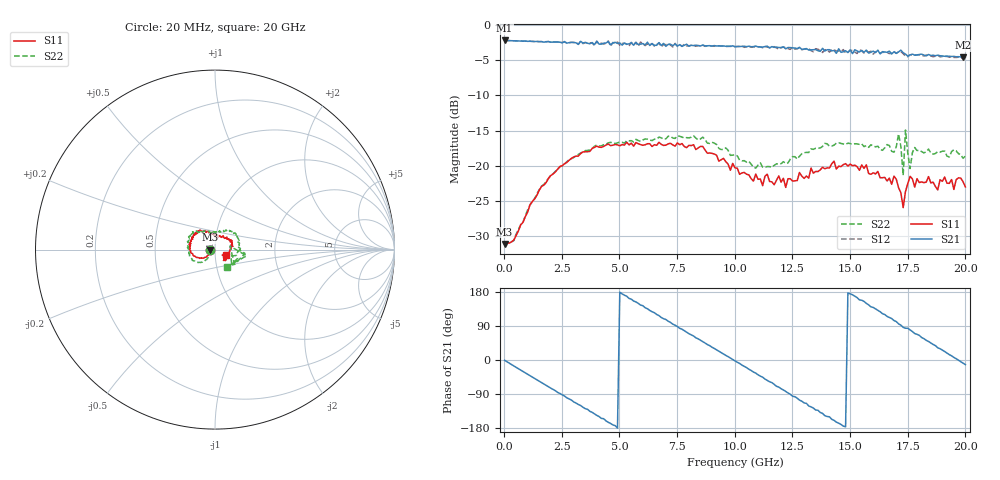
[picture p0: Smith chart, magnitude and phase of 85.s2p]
!Agilent Technologies,N5230A,US43500223,A.07.50.48
!Agilent N5230A: A.07.50.48
!Date: Saturday, September 19, 2015 17:07:46
!Correction: S11(Full 2 Port(1,2))
!S21(Full 2 Port(1,2))
!S12(Full 2 Port(1,2))
!S22(Full 2 Port(1,2))
!S2P File: Measurements: S11, S21, S12, S22:
# Hz S  RI  R 50
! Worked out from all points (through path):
!   201 points, 20 MHz to 20 GHz, reference 50 ohm
!   highest |S21| = -2.19 dB at 20 MHz (marker M1); lowest = -4.6 dB at 19.9 GHz (marker M2)
!   group delay of S21, straight-line fit = 101 ps
!   lowest |S11| = -31.1 dB at 20 MHz (marker M3), VSWR 1.06, Z = 47.3 - j0.034 ohm
!   |S11| at or under -10 dB: start of sweep to end of sweep
!   |S22| runs from -31.4 to -14.9 dB; largest |S21 - S12| = 0.057
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2e7  -0.0278 -0.000359  0.7774 -0.0112  0.7769 -0.0113  -0.0268 0.000192
1.8182e9  -0.0606 -0.0458  0.3007 -0.6992  0.2995 -0.7008  -0.0522 -0.0568
3.4166e9  -0.121 -0.0338  -0.4231 -0.6138  -0.4281 -0.6017  -0.1048 -0.0687
4.9151e9  -0.1398 0.0171  -0.7403 -0.0037  -0.7584 0.00662  -0.1438 -0.022
5.7143e9  -0.141 0.0386  -0.6715 0.3382  -0.6748 0.3387  -0.1536 0.012
6.7133e9  -0.129 0.0702  -0.342 0.6677  -0.346 0.662  -0.1535 0.0451
8.1119e9  -0.0984 0.0984  0.2876 0.6581  0.2739 0.6653  -0.1364 0.0826
9.1109e9  -0.0618 0.1044  0.6162 0.3624  0.6031 0.3704  -0.1016 0.1034
1.001e10  -0.0247 0.0933  0.7017 -0.0291  0.7021 -0.0167  -0.0611 0.1029
1.09091e10  -0.00581 0.0871  0.584 -0.4022  0.5836 -0.3874  -0.0137 0.0954
1.18082e10  0.0127 0.0779  0.2459 -0.6525  0.2617 -0.637  0.0158 0.102
1.34066e10  0.0627 0.0626  -0.3987 -0.5359  -0.3683 -0.5312  0.0828 0.1014
1.5005e10  0.0957 0.0374  -0.6622 0.0645  -0.6635 0.0286  0.1235 0.0735
1.67033e10  0.0791 -0.0205  -0.247 0.6043  -0.2574 0.5722  0.1392 -0.00276
1.71029e10  0.0605 -0.0348  -0.0608 0.642  -0.1018 0.6376  0.1671 -0.0215
1.73027e10  0.04 -0.0307  0.0429 0.6344  0.0201 0.6262  0.0833 0.0195
1.74026e10  0.0526 -0.0392  0.0675 0.6184  0.0428 0.5984  0.1763 -0.0347
1.76024e10  0.0566 -0.0622  0.1143 0.6034  0.0932 0.6079  0.0888 -0.0356
1.78022e10  0.051 -0.0488  0.2113 0.5739  0.1862 0.5818  0.1259 -0.0486
1.83017e10  0.052 -0.0562  0.3725 0.4754  0.354 0.499  0.1016 -0.0743
1.99001e10  0.0676 -0.0367  0.584 -0.0843  0.5772 -0.0629  0.062 -0.0944
2e10  0.0637 -0.031  0.5778 -0.1248  0.5751 -0.1026  0.0676 -0.096
